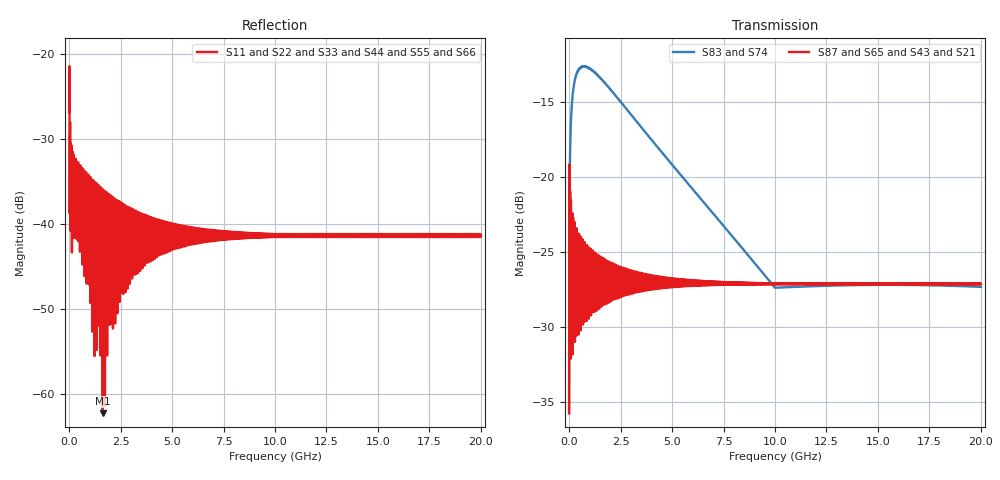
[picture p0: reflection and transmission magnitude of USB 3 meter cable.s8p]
! NPort=8 DATA=2048 NOISE=0 GROUPDELAY=0
! NumOfBlock=1 NumOfParam=0
! .MODEL Smodel S TSTONEFILE=w:\succeed\usb3\models\compliance_sparameters\usb3_spec_compliance_r095_20081106_cable.s8p TYPE=S
! + FBASE=  FMAX=
!  -- The above .MODEL line can be used for the S element in the netlist.
!Port 1-->5
!Port 2-->6
# Hz S RI R  50.0000
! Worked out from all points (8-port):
!   2048 points, 1 kHz to 20 GHz, reference 50 ohm
!   strongest paths, dB at 1 kHz, 5.002 GHz, 10 GHz, 15.01 GHz, 20 GHz:
!     S87: -35.7, -26.8, -27.1, -27.1, -27.1
!     S65: -35.7, -26.8, -27.1, -27.1, -27.1
!     S43: -35.7, -26.8, -27.1, -27.1, -27.1
!     S21: -35.7, -26.8, -27.1, -27.1, -27.1
!     S83: -35.7, -19.2, -27.4, -27.2, -27.3
!     S74: -35.7, -19.2, -27.4, -27.2, -27.3
!   lowest |S11| = -62.3 dB at 1.632 GHz (marker M1), VSWR 1.00, Z = 49.9 + j0.0547 ohm
!   |S11| at or under -10 dB: start of sweep to end of sweep
